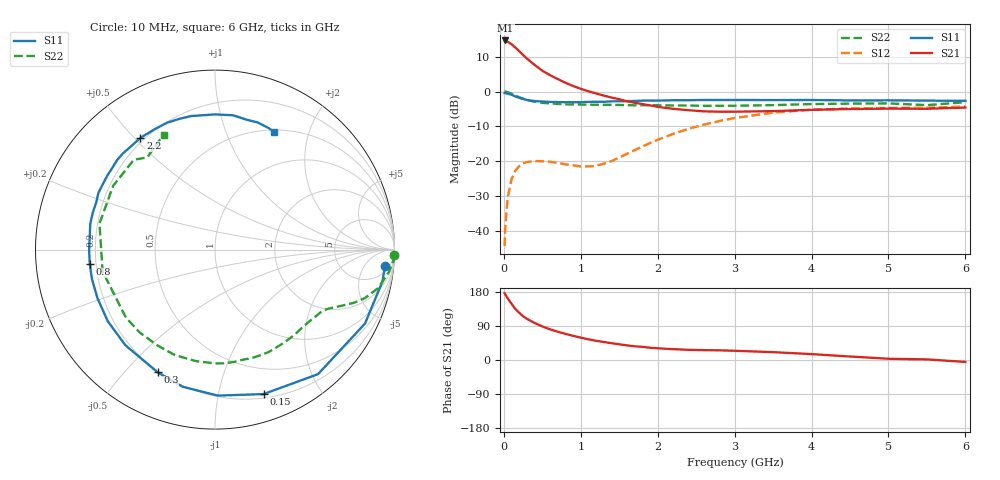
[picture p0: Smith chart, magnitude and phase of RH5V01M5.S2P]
! SIEMENS Small Signal Semiconductors
! BFR106
! Si NPN RF Bipolar Junction Transistor in SOT23
! VCE = 5 V  IC = 1.5 mA
! Common Emitter S-Parameters:  August  1996
# GHz  S  MA  R  50
!  f  S11  S21  S12  S22
! GHz  MAG  ANG  MAG  ANG  MAG  ANG  MAG  ANG
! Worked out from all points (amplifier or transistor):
!   36 points, 10 MHz to 6 GHz, reference 50 ohm
!   highest |S21| = 14.7 dB at 20 MHz (marker M1)
!   |S21| within 3 dB of that: start of sweep to 196.6 MHz
!   unconditionally stable (mu >= 1): 814.4 MHz to 1.843 GHz; 3.579 GHz to end of sweep
!   at 250 MHz: K = 0.29, MSG = 15.6 dB, |S12| = -20.6 dB
!   at 1.4 GHz: K = 1.30, MAG = 5.9 dB, |S12| = -20.0 dB
!   at 6 GHz: K = 1.02, MAG = -1.0 dB, |S12| = -4.3 dB
!   S11 on the Smith chart (normalised r, x): 10 MHz: 8, -16; 150 MHz: 0.24, -1.36; 300 MHz: 0.19, -0.62; 800 MHz: 0.18, -0.06; 2.2 GHz: 0.18, +0.52; 6 GHz: 0.53, +1.49
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0.01  0.952 -5.5  5.382 175.9  0.006 88.1  0.9985 -1.6
0.02  0.9496 -10.8  5.415 173.3  0.012 82.7  0.9988 -3.0
0.05  0.932 -26.2  5.192 162.6  0.0298 75.7  0.9771 -7.3
0.1  0.9006 -50.4  4.78 148.4  0.055 63.2  0.9328 -13.4
0.15  0.8492 -71.4  4.286 134.5  0.073 51.7  0.8768 -18.0
0.2  0.8137 -88.8  3.802 124.6  0.0849 44.4  0.8297 -20.9
0.25  0.7851 -103.3  3.35 115.5  0.0929 37.7  0.7868 -23.1
0.3  0.7548 -115.0  2.974 108.7  0.0971 33.6  0.7561 -24.8
0.4  0.7302 -133.2  2.411 97.7  0.1002 27.2  0.7121 -27.5
0.5  0.7185 -146.2  1.991 88.6  0.0998 23.8  0.6873 -30.0
0.6  0.7087 -157.4  1.717 81.0  0.098 22.5  0.6749 -33.0
0.8  0.7025 -173.4  1.338 69.0  0.0902 25.0  0.6559 -39.3
1.1  0.7098 168.2  1.008 54.6  0.0838 40.5  0.6466 -50.3
1.6  0.7282 145.3  0.724 38.6  0.1271 70.2  0.6383 -70.9
2.2  0.7487 123.7  0.564 28.6  0.2462 71.9  0.6303 -99.7
2.8  0.755 105.2  0.513 25.5  0.3759 59.3  0.6239 -132.3
3.5  0.7534 89.9  0.523 20.7  0.4978 41.5  0.6379 -169.0
4  0.7551 82.3  0.546 15.6  0.5479 29.2  0.6598 167.3
4.5  0.745 76.5  0.56 9.2  0.571 18.6  0.6696 148.0
5  0.7473 71.4  0.568 3.3  0.5818 9.9  0.6748 132.1
5.5  0.7401 66.3  0.565 1.6  0.5843 5.8  0.6375 126.3
6  0.7343 63.2  0.588 -5.1  0.6092 -2.3  0.7024 114.1
